VAR_GLOBAL CONSTANT
	cOversamples 	: UDINT 	:= 10;			// number of oversamples
	cSampleRate		: LREAL		:= 10000.0;		// Samplerate of input signal
	cBufferLength	: UDINT		:= 1600;		// buffer size
	cWindowLength	: UDINT		:= 3200;		// internal buffer size with 50% overlapping
	cFFTResult 		: UDINT 	:= 2049;		// result of mag. spectrum (cFFTLength/2+1)
	cFFTLength		: UDINT		:= 4096;		// length of FFT for mag. spectrum	
	cMaxWindows		: UDINT		:= 3;			// Number of statistic windows
	cChannels		: UDINT		:= 1;			// Number of channels
END_VAR
